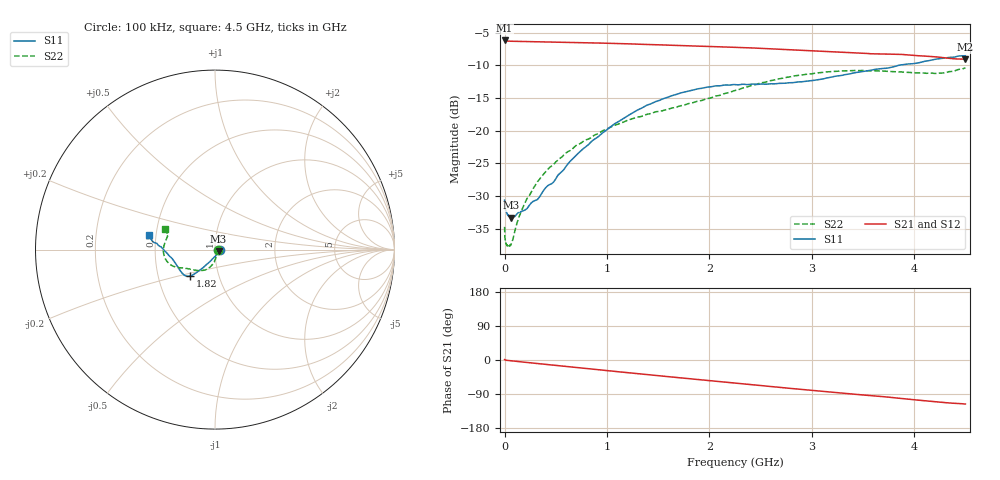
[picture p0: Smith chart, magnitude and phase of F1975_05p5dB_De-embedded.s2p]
! Integrated Device Technology
! Corporate Headquarters
! 6024 Silver Creek Valley Road
! San Jose, CA 95138  USA
! Phone:  1-408-284-8200
! Toll Free:  1-800-223-1366
! Webpage:  http://www.idt.com/
! Timing and RF Division
! 515 Groton Road, Suite 102
! Westford, MA 01886-6024
! Device:  F1975
! Description: 6-bit, 75 ohm, 0.5 dB Digital Step Attenuator
! Frequency:  5.0 MHz -  3.00 GHz
! Package:  4x4 mm QFN Plastic Package: 20 pin
! Ports:  2 RF, 11 DC
!  Pin  1  = D5 (16 dB)
!  Pin  2  = RF1  =  Port 1
!  Pin  3  = Serial Data In (DATA)
!  Pin  4  = Serial Clock (CLK)
!  Pin  5  = Serial Latch Enable (LE)
!  Pin  6  = VDD
!  Pin  7  = NC
!  Pin  8  = NC
!  Pin  9  = NC
!  Pin 10  = GND
!  Pin 11  = GND
!  Pin 12  = NC
!  Pin 13  = VMODE
!  Pin 14  = RF2  =  Port 2
!  Pin 15  = D4 (8 dB)
!  Pin 16  = D3 (4 dB)
!  Pin 17  = D2 (2 dB)
!  Pin 18  = NC
!  Pin 19  = D1 (1 dB)
!  Pin 20  = D0 (0.5 dB)
! State:  11
! Atten State:  5.5 dB
! Voltage:  +3.30 Volts
! Current:  0.564 mA
! Data:  The device was measured on a F1975 evaluation board which has
!  individual transmission lines to the RF pins.  Data was collected
!  using a calibrated network analyzer.  The evaluation board was
!  de-embedded using Automatic Fixture Removal (AFR).
!  The reference plane is the edge of the package pin.
! Misc:
!  Action Tracker AT0415
! Date Measured:  2018-02-08
! Date:  2018-03-26  MJV
! Note:
!  Integrated Device Technology supplies this data as a sample of measured
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# GHz S dB R 75
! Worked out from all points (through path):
!   291 points, 100 kHz to 4.5 GHz, reference 75 ohm
!   highest |S21| = -6.21 dB at 100 kHz (marker M1); lowest = -9.1 dB at 4.5 GHz (marker M2)
!   group delay of S21, straight-line fit = 72.7 ps
!   lowest |S11| = -33.3 dB at 60 MHz (marker M3), VSWR 1.04, Z = 78 - j1.29 ohm
!   |S11| at or under -10 dB: start of sweep to 3.853 GHz
!   |S22| runs from -37.7 to -10.4 dB; largest |S21 - S12| = 0.00019
!   S11 on the Smith chart (normalised r, x): 100 kHz: 1.06, +0.00; 1.82 GHz: 0.73, -0.22; 4.5 GHz: 0.46, +0.08
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0.0001  -30.63 0.1  -6.21 1.2  -6.21 1.2  -34.70 0.1
0.0009  -31.38 -2.5  -6.24 1.0  -6.24 1.0  -35.80 -2.8
0.002  -31.71 -2.7  -6.26 0.8  -6.26 0.8  -36.23 -4.0
0.013  -32.30 -8.2  -6.29 -0.6  -6.29 -0.6  -37.22 -15.2
0.022  -32.64 -10.2  -6.30 -0.9  -6.30 -0.9  -37.58 -21.7
0.06  -33.33 -22.5  -6.33 -2.0  -6.33 -2.0  -37.50 -43.7
0.16  -32.38 -45.9  -6.38 -4.9  -6.38 -4.9  -32.43 -71.1
0.22  -31.90 -58.5  -6.39 -6.5  -6.39 -6.5  -30.34 -76.1
0.26  -31.05 -65.1  -6.41 -7.6  -6.41 -7.7  -29.40 -79.6
0.32  -30.53 -74.0  -6.43 -9.3  -6.42 -9.3  -27.82 -83.0
0.4  -28.74 -85.2  -6.45 -11.5  -6.45 -11.5  -26.29 -85.6
0.5  -27.36 -96.9  -6.48 -14.2  -6.48 -14.2  -24.78 -89.9
0.76  -22.87 -112.4  -6.56 -21.4  -6.56 -21.4  -21.73 -98.7
1.08  -18.90 -122.3  -6.67 -30.2  -6.67 -30.2  -19.15 -108.8
1.52  -15.32 -129.5  -6.88 -41.9  -6.88 -41.9  -17.03 -124.0
1.82  -13.87 -133.4  -7.05 -49.7  -7.05 -49.7  -15.78 -135.5
2.26  -12.96 -142.7  -7.27 -61.1  -7.27 -61.1  -13.83 -149.4
2.68  -12.77 -156.2  -7.54 -72.0  -7.54 -72.0  -12.08 -157.9
3.02  -12.31 -167.5  -7.80 -80.6  -7.80 -80.6  -11.25 -165.7
3.76  -10.38 176.9  -8.31 -98.3  -8.30 -98.3  -10.95 174.1
4.22  -9.05 172.2  -8.73 -110.5  -8.73 -110.5  -11.25 162.2
4.5  -8.55 167.7  -9.07 -116.2  -9.07 -116.2  -10.39 158.1
